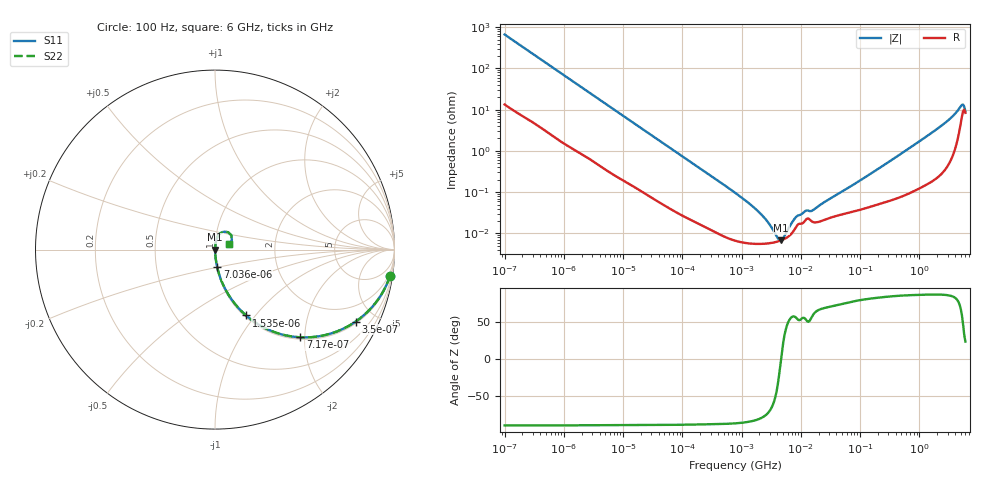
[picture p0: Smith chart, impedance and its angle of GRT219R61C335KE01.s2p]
!Murata Part Number: GRT219R61C335KE01
!These Parameters are Measured in Series Mode Connection
!Data Generated on Jun 19, 2026
!  o--ll--o
!Port1  Port2
!  o------o
!Operation Temp=25[degC], DC Bias Voltage=0[V]
!Freq. Start=100[Hz] Stop=6[GHz] 401[Steps]
# Hz S RI R 50
!Freq.(Hz) S11(Real) S11(Imag) S21(Real) S21(Imag) S12(Real) S12(Imag) S22(Real) S22(Imag)
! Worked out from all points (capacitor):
!   401 points, 100 Hz to 6 GHz, reference 50 ohm
!   read as one part in series: C = 2.39 uF near 109 Hz
!   lowest |Z| = 6.77 mohm at 4.644 MHz (marker M1)
!   series resonance near 4.639 MHz, so ESL is about 490 pH
!   S11 on the Smith chart (normalised r, x): 100 Hz: 1, -13; 350 Hz: 1.08, -3.86; 717 Hz: 1.04, -1.90; 1.535 kHz: 1.02, -0.90; 7.036 kHz: 1.01, -0.20; 6 GHz: 1.17, +0.07
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100  0.975 -0.1463  0.025 0.1463  0.025 0.1463  0.975 -0.1463
205  0.9099 -0.276  0.0901 0.276  0.0901 0.276  0.9099 -0.276
350  0.783 -0.4014  0.217 0.4014  0.217 0.4014  0.783 -0.4014
717  0.4758 -0.4886  0.5242 0.4886  0.5242 0.4886  0.4758 -0.4886
1535  0.1734 -0.3671  0.8266 0.3671  0.8266 0.3671  0.1734 -0.3671
2008  0.1119 -0.3034  0.8881 0.3034  0.8881 0.3034  0.1119 -0.3034
7036  0.0125 -0.0988  0.9875 0.0988  0.9875 0.0988  0.0125 -0.0988
40335  0.000895 -0.018  0.9991 0.018  0.9991 0.018  0.000895 -0.018
774597  6.76e-05 -0.000969  0.9999 0.000969  0.9999 0.000969  6.76e-05 -0.000969
1983483  5.57e-05 -0.00032  0.9999 0.00032  0.9999 0.00032  5.57e-05 -0.00032
3712478  6.14e-05 -7.56e-05  0.9999 7.56e-05  0.9999 7.56e-05  6.14e-05 -7.56e-05
4643984  6.77e-05 4e-07  0.9999 -4e-07  0.9999 -4e-07  6.77e-05 4e-07
5554849  7.63e-05 6.2e-05  0.9999 -6.2e-05  0.9999 -6.2e-05  7.63e-05 6.2e-05
8692127  0.000157 0.000213  0.9998 -0.000213  0.9998 -0.000213  0.000157 0.000213
1.189169e7  0.000206 0.000282  0.9998 -0.000282  0.9998 -0.000282  0.000206 0.000282
1.555665e7  0.000193 0.0003  0.9998 -0.0003  0.9998 -0.0003  0.000193 0.0003
3.124326e8  0.000642 0.00549  0.9994 -0.00549  0.9994 -0.00549  0.000642 0.00549
2.34314e9  0.00433 0.04  0.9957 -0.04  0.9957 -0.04  0.00433 0.04
3.505958e9  0.0106 0.0638  0.9894 -0.0638  0.9894 -0.0638  0.0106 0.0638
5.016141e9  0.0555 0.1001  0.9445 -0.1001  0.9445 -0.1001  0.0555 0.1001
5.245841e9  0.0738 0.0962  0.9262 -0.0962  0.9262 -0.0962  0.0738 0.0962
6e9  0.0783 0.0306  0.9217 -0.0306  0.9217 -0.0306  0.0783 0.0306
